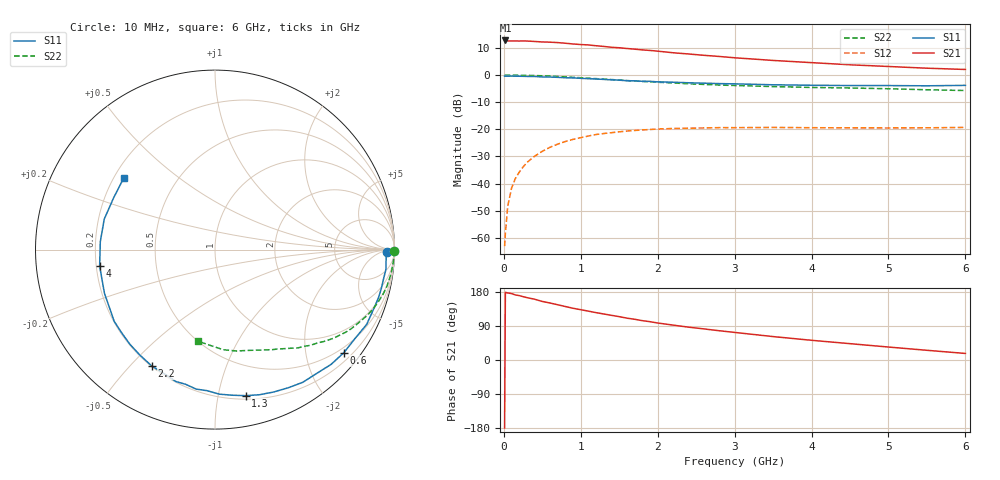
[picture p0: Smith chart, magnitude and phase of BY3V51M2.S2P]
! SIEMENS Small Signal Semiconductors
! BFY420
! Si NPN RF SIEGET Grounded Emitter Transistor in MICRO-X
! VCE = 3.5 V  IC = 1.2 mA
! Common Emitter S-Parameters:  October  1996
# GHz  S  MA  R  50
!  f  S11  S21  S12  S22
! GHz  MAG  ANG  MAG  ANG  MAG  ANG  MAG  ANG
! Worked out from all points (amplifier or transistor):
!   36 points, 10 MHz to 6 GHz, reference 50 ohm
!   highest |S21| = 12.8 dB at 20 MHz (marker M1)
!   |S21| within 3 dB of that: start of sweep to 1.614 GHz
!   unconditionally stable (mu >= 1): 4.389 GHz to end of sweep
!   at 250 MHz: K = 0.05, MSG = 23.2 dB, |S12| = -33.9 dB
!   at 1.4 GHz: K = 0.21, MSG = 15.8 dB, |S12| = -21.2 dB
!   at 6 GHz: K = 1.30, MAG = 7.4 dB, |S12| = -19.3 dB
!   S11 on the Smith chart (normalised r, x): 10 MHz: 41, -11; 600 MHz: 0.38, -2.80; 1.3 GHz: 0.23, -1.21; 2.2 GHz: 0.20, -0.58; 4 GHz: 0.21, -0.07; 6 GHz: 0.24, +0.33
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0.01  0.9559 -0.7  4.339 -179.4  0.0007 59.9  0.9988 -0.4
0.02  0.955 -1.5  4.349 178.6  0.0012 75.9  0.9999 -0.7
0.05  0.9549 -3.3  4.266 176.9  0.0038 83.4  0.9972 -1.5
0.1  0.9587 -6.6  4.264 175.3  0.0082 85.9  0.9966 -3.0
0.15  0.9532 -9.7  4.258 171.7  0.0124 81.8  0.9949 -4.6
0.2  0.9517 -13.2  4.244 170.0  0.0162 81.8  0.9926 -5.9
0.3  0.9451 -19.4  4.246 164.6  0.0245 79.0  0.9867 -9.0
0.4  0.9423 -26.2  4.168 160.4  0.0319 74.4  0.9795 -12.0
0.5  0.9242 -32.4  4.081 154.5  0.0393 71.1  0.9691 -14.8
0.6  0.9193 -38.7  4.043 150.4  0.0466 67.4  0.9557 -17.6
0.8  0.8929 -50.5  3.865 141.1  0.0596 60.0  0.926 -23.1
1.1  0.858 -67.7  3.594 128.9  0.0753 50.7  0.8773 -30.2
1.3  0.8317 -78.1  3.372 121.4  0.0837 45.1  0.8421 -34.5
1.6  0.7873 -93.2  3.091 110.4  0.0928 37.7  0.7924 -40.3
1.8  0.7681 -102.3  2.914 103.8  0.0972 33.4  0.7638 -43.5
2.2  0.738 -118.5  2.579 92.1  0.1036 25.9  0.716 -49.9
2.8  0.6964 -138.5  2.205 77.2  0.1074 17.8  0.655 -57.7
3.5  0.6622 -158.5  1.862 61.8  0.1082 11.9  0.6137 -65.8
4  0.6492 -171.9  1.696 52.0  0.1071 9.0  0.5914 -71.7
4.5  0.6405 176.1  1.548 43.1  0.1063 7.1  0.5776 -78.0
5.5  0.6342 153.0  1.339 25.6  0.1066 6.7  0.5359 -92.3
6  0.646 142.0  1.269 17.3  0.1083 7.3  0.5189 -100.5
